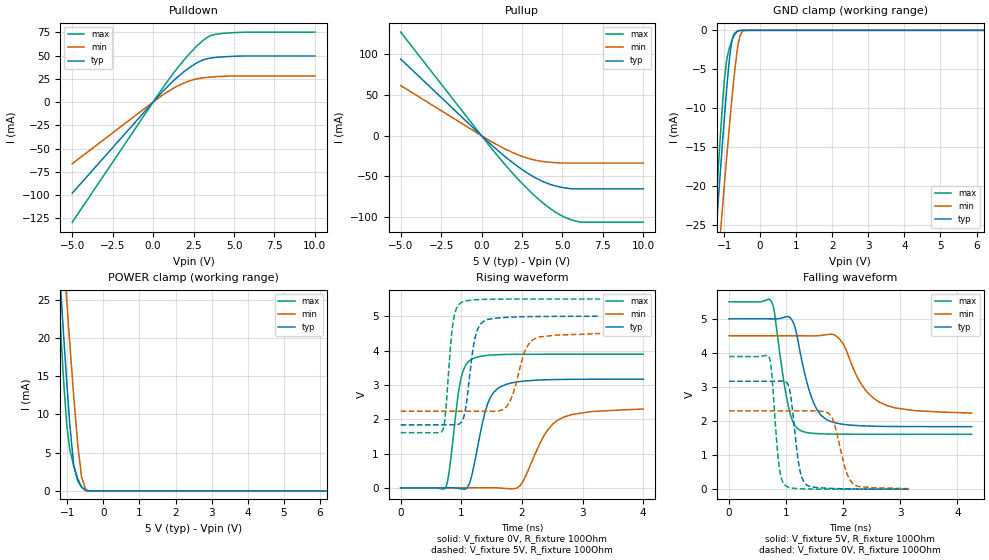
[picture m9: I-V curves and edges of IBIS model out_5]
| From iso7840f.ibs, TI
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|   out_5 Model
[Model]   out_5
Model_type   3-state
Polarity   Non-Inverting
Vmeas = 2.5
Vref = 0
Cref = 15pF
Rref = 150
|   typ   min   max
|   (nom PVT)   (fast PVT)   (slow PVT)
C_comp   9.635e-13   9.413e-13   9.787e-13
| Where nom  PVT is Nominal Process, 5V, 27C
|   Fast PVT is Strong Process,  5.5V, -55C
|   Slow PVT is Weak Process,   4.5V, 150C
[Voltage Range]   5   4.5   5.5
|Junction Temperature
[Temperature Range]   27   150   -55
[Pullup Reference]   5   4.5   5.5
[Pulldown Reference]   0   0   0
[Power Clamp Reference]   5   4.5   5.5
[GND Clamp Reference]   0   0   0
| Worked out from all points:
|   slope of the pulldown table from 0 to 0.75 V, typ, clamps not added: 52.8 ohm
|   slope of the pullup table from 0 to 0.75 V, typ, clamps not added: 54.8 ohm
|   GND clamp passes 1 mA (typ) near -0.76 V on its own axis
|   POWER clamp passes 1 mA (typ) near -0.67 V on its own axis
|   falling waveform, V_fixture 5V, R_fixture 100Ohm: 20-80 % time 294ps typ, 457ps min, 213ps max; typ from 5 V to 1.83 V
|   rising waveform, V_fixture 0V, R_fixture 100Ohm: 20-80 % time 247ps typ, 408ps min, 166ps max; typ from 0 V to 3.17 V
|   rising waveform, V_fixture 5V, R_fixture 100Ohm: 20-80 % time 143ps typ, 221ps min, 107ps max; typ from 1.83 V to 5 V
|   falling waveform, V_fixture 0V, R_fixture 100Ohm: 20-80 % time 137ps typ, 206ps min, 108ps max; typ from 3.17 V to 0.001 V
[Pulldown]
|   Voltage   I(typ)   I(min)   I(max)
-5V       -97.96mA   -66.29mA   -129.3mA
700mV     13.33mA    8.861mA    17.83mA
1.3V      23.59mA    15.28mA    32.05mA
1.97V     33.54mA    20.95mA    46.53mA
2.663V    41.75mA    24.82mA    59.55mA
3.096V    45.35mA    26.09mA    66.4mA
3.591V    47.4mA     26.94mA    71.64mA
4.416V    48.75mA    27.74mA    74.07mA
5.912V    49.52mA    28.03mA    75.26mA
10V       49.52mA    28.03mA    75.26mA
[GND Clamp]
|   Voltage   I(typ)   I(min)   I(max)
-5V       -291.7mA   -259.7mA   -341.9mA
-1.469V   -42.36mA   -47.38mA   -41.81mA
-1.2V     -24.34mA   -31.61mA   -20.61mA
-1.101V   -17.93mA   -25.94mA   -13.29mA
-1.026V   -13.29mA   -21.76mA   -8.356mA
-940mV    -8.166mA   -16.97mA   -4.222mA
-810.5mV  -2.106mA   -10.13mA   -1.616mA
-737.5mV  -623.1uA   -6.594mA   -788.2uA
-638.5mV  -109.1uA   -2.6mA     -169uA
-558.5mV  -21.67uA   -689.5uA   -27.72uA
-387.5mV  -336nA     -9.718uA   -155.2nA
10V       0A         0A         0A
[Pullup]
|   Voltage   I(typ)   I(min)   I(max)
-5V       94.16mA    61.66mA    127.2mA
100mV     -1.88mA    -1.233mA   -2.555mA
1.3V      -23.12mA   -14.74mA   -31.91mA
2.753V    -44.75mA   -26.97mA   -63.54mA
3.883V    -57.04mA   -31.9mA    -83.94mA
4.338V    -60.4mA    -32.77mA   -90.72mA
4.935V    -63.28mA   -33.6mA    -97.99mA
5.49V     -64.99mA   -33.6mA    -102.8mA
5.984V    -65.24mA   -33.6mA    -105.5mA
10V       -65.24mA   -33.6mA    -106.2mA
[POWER Clamp]
|   Voltage   I(typ)   I(min)   I(max)
-5V       516mA      373mA      669.1mA
-1.535V   53.28mA    61.23mA    50.65mA
-1.128V   22.12mA    32.46mA    16.25mA
-1.101V   20.12mA    30.56mA    14.17mA
-1.018V   14.26mA    24.94mA    8.698mA
-935.5mV  8.857mA    19.46mA    5.475mA
-825mV    3.399mA    12.45mA    3.258mA
-710mV    1.283mA    5.971mA    1.578mA
-608mV    501.8uA    1.883mA    547.9uA
-500mV    100.1uA    287.4uA    70.26uA
-260mV    196.4nA    1.991uA    20.04nA
10V       0A         0A         0A
[Ramp]
R_load = 100
|   typ   min   max
dV/dt_r   1.89957/2.46376e-10   1.37816/4.05923e-10   2.33584/1.64284e-10
dV/dt_f   1.89917/2.94008e-10   1.35969/4.56241e-10   2.33391/2.13444e-10
[Falling Waveform]
V_fixture = 5V
V_fixture_min = 4.5V
V_fixture_max = 5.5V
R_fixture = 100Ohm
|   Time   V(typ)   V(min)   V(max)
0s        5V         4.5V       5.5V
744ps     4.998V     4.5V       5.503V
794ps     4.997V     4.5V       5.211V
1.044ns   5.061V     4.5V       2.402V
1.138ns   4.843V     4.5V       1.919V
1.248ns   3.995V     4.5V       1.724V
1.508ns   2.44V      4.498V     1.634V
1.788ns   1.982V     4.55V      1.617V
2.632ns   1.844V     2.556V     1.61V
4.25ns    1.835V     2.234V     1.61V
[Rising Waveform]
V_fixture = 0V
V_fixture_min = 0V
V_fixture_max = 0V
R_fixture = 100Ohm
|   Time   V(typ)   V(min)   V(max)
0s        9.106nV    157nV      6.985nV
744ps     604.6uV    260.4nV    13.64mV
802ps     2.16mV     1.688uV    505.1mV
996ps     -28.61mV   2.652uV    3.192V
1.182ns   430.5mV    -87.19uV   3.759V
1.394ns   2.227V     1.211mV    3.854V
1.62ns    2.92V      -2.79mV    3.881V
1.966ns   3.096V     58.8mV     3.89V
2.586ns   3.157V     1.967V     3.893V
4ns       3.166V     2.297V     3.893V
[Rising Waveform]
V_fixture = 5V
V_fixture_min = 4.5V
V_fixture_max = 5.5V
R_fixture = 100Ohm
|   Time   V(typ)   V(min)   V(max)
0s        1.834V     2.233V     1.608V
694ps     1.834V     2.233V     1.686V
738ps     1.835V     2.233V     2.144V
862ps     1.836V     2.233V     4.793V
1.002ns   1.916V     2.233V     5.4V
1.234ns   4.427V     2.233V     5.479V
1.366ns   4.853V     2.233V     5.49V
1.78ns    4.97V      2.451V     5.499V
2.204ns   4.991V     4.338V     5.5V
3.29ns    5V         4.499V     5.5V
[Falling Waveform]
V_fixture = 0V
V_fixture_min = 0V
V_fixture_max = 0V
R_fixture = 100Ohm
|   Time   V(typ)   V(min)   V(max)
0s        3.167V     2.298V     3.895V
702ps     3.166V     2.298V     3.871V
864ps     3.168V     2.298V     859.2mV
982ps     3.161V     2.298V     114.4mV
1.07ns    2.85V      2.298V     41.6mV
1.246ns   519.4mV    2.297V     11.36mV
1.364ns   117.4mV    2.297V     5.057mV
1.794ns   22.18mV    2.137V     335.4uV
2.2ns     7.039mV    126.4mV    43.09uV
3.152ns   812.6uV    15.03mV    527nV
